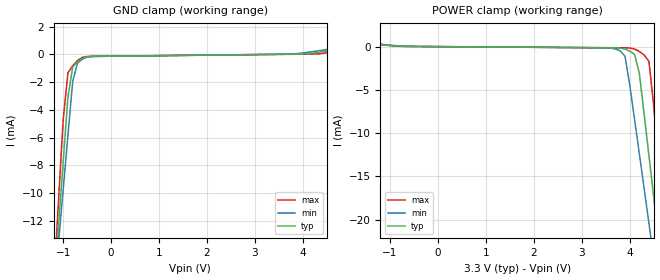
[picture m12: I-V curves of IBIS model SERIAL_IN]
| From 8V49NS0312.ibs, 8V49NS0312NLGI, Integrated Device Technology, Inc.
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[Model] SERIAL_IN
Model_type   Input
Polarity   Non-Inverting
|   typ   min   max
C_comp   2pF   1.5pF   2.5pF
|Input
Vinl = 0.8V
Vinh = 2.0V
|   typ   min   max
[Voltage range]   3.3V   3.135V   3.465V
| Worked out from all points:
|   GND clamp passes 1 mA (typ) near -0.80 V on its own axis
|   POWER clamp passes 1 mA (typ) near -2.33 V on its own axis
[GND_clamp]
|Voltage   I (typ)   I (min)   I (max)
|Note, modeling breaks down at 250mA and above.  This is well beyond the functional   |
|operating range of the device.  Should this scenario occur, catastrophic failure and   |
|possible damage to the device and/or board is of higher concern than the I-V curve   |
|behavior.  The IBIS checker will flag currents in excess of 10A with warnings.  Lines   |
|with currents in excess of 0.35 A have been commented out.  The points still remain|
|available to the user if the user desires to use them.   |
-3.3V     -120.1mA   -104.4mA   -146.1mA
-1.2V     -17.4mA    -17.85mA   -16.9mA
-1.1V     -12.6mA    -13.82mA   -10.82mA
-1V       -7.826mA   -9.83mA    -4.78mA
-900mV    -3.097mA   -5.869mA   -1.329mA
-800mV    -907.8uA   -1.951mA   -813.2uA
-700mV    -522.7uA   -626.2uA   -443.8uA
-600mV    -283.7uA   -342.2uA   -218.1uA
-400mV    -146.1uA   -152.2uA   -139.6uA
3.7V      15.58uA    25.41uA    8.474uA
4.3V      144.3uA    253.7uA    37.42uA
6.6V      1.656mA    1.582mA    1.788mA
[Power_clamp]
|Voltage   I (typ)   I (min)   I (max)
|Note, modeling breaks down at 250mA and above.  This is well beyond the functional   |
|operating range of the device.  Should this scenario occur, catastrophic failure and   |
|possible damage to the device and/or board is of higher concern than the I-V curve   |
|behavior.  The IBIS checker will flag currents in excess of 10A with warnings.  Lines   |
|with currents in excess of 0.35 A have been commented out.  The points still remain|
|available to the user if the user desires to use them.   |
-3.3V     1.656mA    1.484mA    1.923mA
-900mV    93.8uA     123.4uA    58.06uA
3.7V      -146.1uA   -277.6uA   -133.4uA
3.9V      -283.7uA   -1.11mA    -141.5uA
4.1V      -907.8uA   -8.4mA     -277.5uA
4.2V      -3.097mA   -12.38mA   -559.4uA
4.4V      -12.6mA    -20.43mA   -1.708mA
4.5V      -17.4mA    -24.48mA   -6.891mA
4.6V      -22.22mA   -28.55mA   -12.95mA
4.7V      -27.05mA   -32.63mA   -19.03mA
4.8V      -31.9mA    -36.72mA   -25.14mA
6.6V      -120.1mA   -111.3mA   -135.9mA
